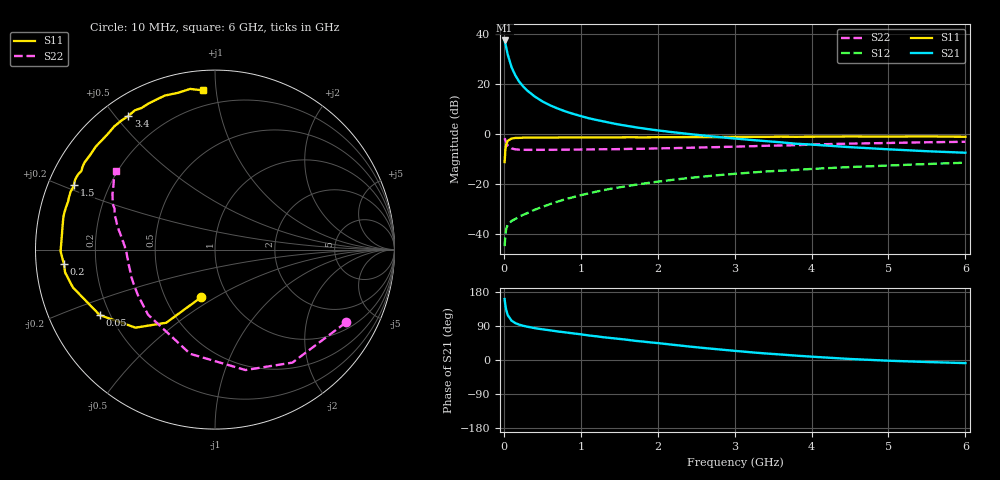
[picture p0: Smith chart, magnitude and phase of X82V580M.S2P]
! SIEMENS Small Signal Semiconductors
! BFP136W
! Si NPN RF Bipolar Junction Transistor in SOT343
! VCE = 2.5 V  IC = 80 mA
! Common Emitter S-Parameters:  September  1994
# GHz  S  MA  R  50
!  f  S11  S21  S12  S22
! GHz  MAG  ANG  MAG  ANG  MAG  ANG  MAG  ANG
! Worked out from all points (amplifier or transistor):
!   40 points, 10 MHz to 6 GHz, reference 50 ohm
!   highest |S21| = 37.5 dB at 10 MHz (marker M1)
!   |S21| within 3 dB of that: start of sweep to 32.17 MHz
!   unconditionally stable (mu >= 1): 516.3 MHz to 2.909 GHz
!   at 200 MHz: K = 0.66, MSG = 27.0 dB, |S12| = -32.9 dB
!   at 1.5 GHz: K = 1.11, MAG = 10.5 dB, |S12| = -21.2 dB
!   at 6 GHz: K = 0.97, MSG = 2.0 dB, |S12| = -11.4 dB
!   S11 on the Smith chart (normalised r, x): 10 MHz: 0.75, -0.43; 50 MHz: 0.16, -0.26; 200 MHz: 0.08, -0.05; 1.5 GHz: 0.08, +0.22; 3.4 GHz: 0.08, +0.54; 6 GHz: 0.11, +0.92
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0.01  0.2779 -106.4  74.86 160.8  0.0058 70.8  0.8348 -29.1
0.02  0.4898 -123.7  64.76 144.6  0.0096 57.4  0.7631 -55.6
0.03  0.6205 -135.5  54.93 132.9  0.0127 48.9  0.6922 -75.8
0.05  0.7386 -150.4  39.48 118.7  0.0155 39.4  0.597 -103.4
0.1  0.8194 -165.1  21.92 103.8  0.0185 34.9  0.5203 -135.9
0.15  0.8447 -171.3  14.94 97.3  0.0203 38.1  0.4987 -149.6
0.2  0.8455 -174.7  11.22 93.3  0.0226 40.2  0.4921 -157.0
0.25  0.8547 -177.7  9.053 90.3  0.0245 42.7  0.4903 -161.8
0.3  0.8605 -179.4  7.565 88.1  0.0263 45.9  0.4876 -165.0
0.4  0.857 176.9  5.7 84.2  0.031 50.5  0.4877 -169.3
0.5  0.8569 174.4  4.545 81.0  0.0353 53.7  0.4883 -172.1
0.6  0.8583 172.3  3.792 78.4  0.0401 55.5  0.489 -174.0
0.7  0.8607 169.9  3.268 75.3  0.0451 58.1  0.4908 -175.3
0.9  0.864 166.3  2.558 70.2  0.0552 59.7  0.4929 -177.9
1.1  0.8613 161.8  2.095 64.8  0.0658 60.5  0.497 -179.5
1.5  0.8651 155.4  1.559 55.7  0.0868 60.0  0.5048 177.4
2.2  0.8727 143.0  1.096 40.2  0.123 55.3  0.5274 172.1
3.2  0.888 126.1  0.773 20.6  0.1707 46.0  0.5753 163.3
3.4  0.8873 123.0  0.73 17.3  0.18 43.9  0.5886 161.4
4.5  0.9027 108.1  0.552 2.7  0.2209 33.7  0.65 151.5
5.5  0.9058 98.8  0.458 -5.3  0.2541 25.7  0.6913 144.5
6  0.89 94.4  0.427 -8.2  0.2703 21.3  0.707 141.5
